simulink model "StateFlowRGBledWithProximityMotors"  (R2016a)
settings: Solver=FixedStepAuto  StartTime=0.0  StopTime=inf  RelTol=1e-3
libraries: miniQ x3

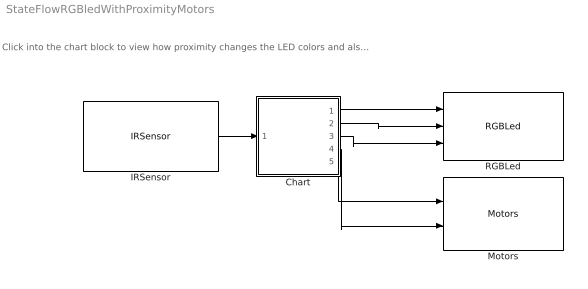
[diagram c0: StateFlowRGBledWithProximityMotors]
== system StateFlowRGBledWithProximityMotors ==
  note: Click into the chart block to view how proximity changes the LED colors and also the motor direction
  Chart : Stateflow chart  TreatAsAtomicUnit=on
  IRSensor : miniQ/IRSensor  sampleTime_dd=0.01  debug_dd=off
  Motors : miniQ/Motors  flipLeft=off  flipRight=off
  RGBLed : miniQ/RGBLed
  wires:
  IRSensor/1 -> Chart/1(prox)
  Chart/1(r) -> RGBLed/1
  Chart/2(g) -> RGBLed/2
  Chart/3(b) -> RGBLed/3
  Chart/4(MR) -> Motors/2
  Chart/5(ML) -> Motors/1

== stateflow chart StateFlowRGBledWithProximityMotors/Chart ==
  state Green
    entry: r=0;
    g=255;
    b=0;
    MR=255;
    ML=255;
  state No object = green light [group]
  state Red
    entry: r = 255;
    g=0;
    b=0;
    MR=-255;
    ML=255;
  state Object detected = red light [group]
  (default) -> Green
  Green -> Red : [prox>10]
  Red -> Green : [prox<10]
  data: prox input; r output; g output; b output; MR output; ML output
